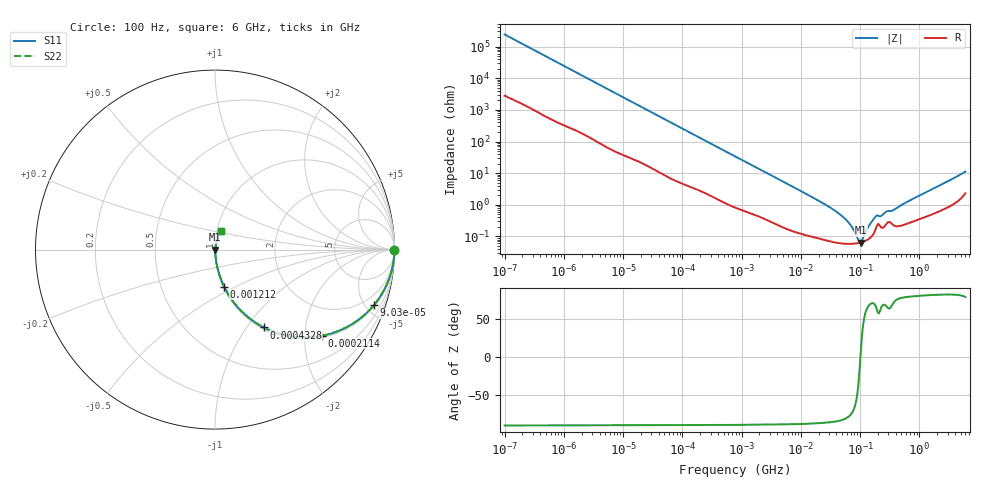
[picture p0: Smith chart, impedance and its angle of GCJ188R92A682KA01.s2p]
!Murata Part Number: GCJ188R92A682KA01
!These Parameters are Measured in Series Mode Connection
!Data Generated on Mar 13, 2026
!  o--ll--o
!Port1  Port2
!  o------o
!Operation Temp=25[degC], DC Bias Voltage=0[V]
!Freq. Start=100[Hz] Stop=6[GHz] 401[Steps]
# Hz S RI R 50
!Freq.(Hz) S11(Real) S11(Imag) S21(Real) S21(Imag) S12(Real) S12(Imag) S22(Real) S22(Imag)
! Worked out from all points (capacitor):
!   401 points, 100 Hz to 6 GHz, reference 50 ohm
!   read as one part in series: C = 6.59 nF near 109 Hz
!   lowest |Z| = 64.5 mohm at 102 MHz (marker M1)
!   series resonance near 101.4 MHz, so ESL is about 370 pH
!   S11 on the Smith chart (normalised r, x): 100 Hz: open; 90.3 kHz: 1.10, -5.67; 211.4 kHz: 1.05, -2.45; 432.8 kHz: 1.03, -1.21; 1.212 MHz: 1.01, -0.44; 6 GHz: 1.05, +0.22
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100  1 -0.000415  5e-06 0.000415  5e-06 0.000415  1 -0.000415
2008  0.9998 -0.00814  0.000186 0.00814  0.000186 0.00814  0.9998 -0.00814
12592  0.9967 -0.05  0.0033 0.05  0.0033 0.05  0.9967 -0.05
40335  0.973 -0.154  0.027 0.154  0.027 0.154  0.973 -0.154
90302  0.8851 -0.3102  0.1149 0.3102  0.1149 0.3102  0.8851 -0.3102
211427  0.5976 -0.4797  0.4024 0.4797  0.4024 0.4797  0.5976 -0.4797
432798  0.272 -0.4339  0.728 0.4339  0.728 0.4339  0.272 -0.4339
774597  0.1093 -0.3002  0.8907 0.3002  0.8907 0.3002  0.1093 -0.3002
1212075  0.0507 -0.2062  0.9493 0.2062  0.9493 0.2062  0.0507 -0.2062
3549919  0.0083 -0.0753  0.9917 0.0753  0.9917 0.0753  0.0083 -0.0753
1.555665e7  0.00128 -0.0174  0.9987 0.0174  0.9987 0.0174  0.00128 -0.0174
3.330331e7  0.000737 -0.00757  0.9993 0.00757  0.9993 0.00757  0.000737 -0.00757
5.211241e7  0.000609 -0.00404  0.9994 0.00404  0.9994 0.00404  0.000609 -0.00404
6.817316e7  0.000587 -0.00231  0.9994 0.00231  0.9994 0.00231  0.000587 -0.00231
9.326766e7  0.00062 -0.000481  0.9994 0.000481  0.9994 0.000481  0.00062 -0.000481
1.020051e8  0.000644 3.25e-05  0.9994 -3.25e-05  0.9994 -3.25e-05  0.000644 3.25e-05
1.115611e8  0.000677 0.000552  0.9993 -0.000552  0.9993 -0.000552  0.000677 0.000552
1.395531e8  0.000832 0.00193  0.9992 -0.00193  0.9992 -0.00193  0.000832 0.00193
1.745687e8  0.00138 0.00356  0.9986 -0.00356  0.9986 -0.00356  0.00138 0.00356
3.124326e8  0.00291 0.00565  0.9971 -0.00565  0.9971 -0.00565  0.00291 0.00565
3.737127e8  0.00226 0.00658  0.9977 -0.00658  0.9977 -0.00658  0.00226 0.00658
6e9  0.0338 0.1035  0.9662 -0.1035  0.9662 -0.1035  0.0338 0.1035
